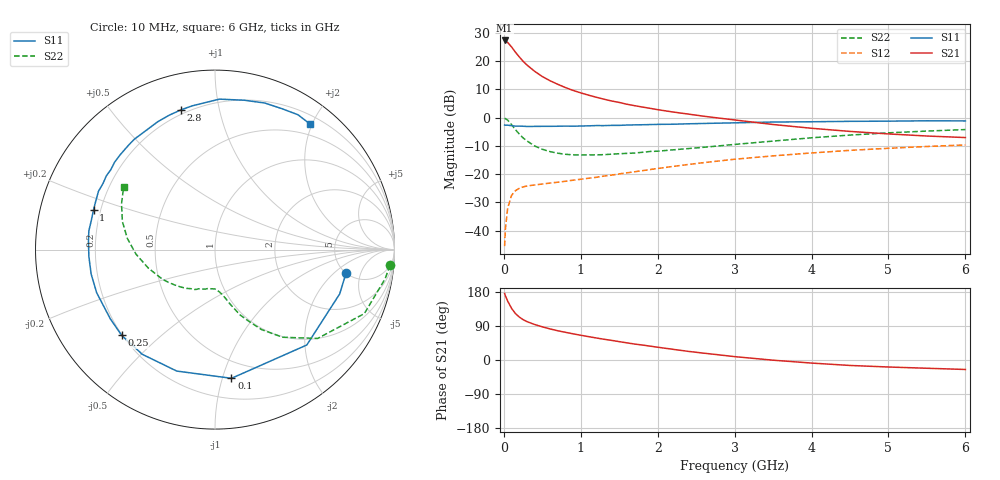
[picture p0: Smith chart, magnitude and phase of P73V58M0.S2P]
! SIEMENS Small Signal Semiconductors
! BFP196
! Si NPN RF Bipolar Junction Transistor in SOT143
! VCE = 3.5 V  IC = 8 mA
! Common Emitter S-Parameters:  May  1996
# GHz  S  MA  R  50
!  f  S11  S21  S12  S22
! GHz  MAG  ANG  MAG  ANG  MAG  ANG  MAG  ANG
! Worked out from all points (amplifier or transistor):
!   36 points, 10 MHz to 6 GHz, reference 50 ohm
!   highest |S21| = 27.4 dB at 10 MHz (marker M1)
!   |S21| within 3 dB of that: start of sweep to 119.2 MHz
!   unconditionally stable (mu >= 1): 947.1 MHz to 3.184 GHz
!   at 250 MHz: K = 0.34, MSG = 22.3 dB, |S12| = -24.5 dB
!   at 1.4 GHz: K = 1.15, MAG = 10.8 dB, |S12| = -20.3 dB
!   at 6 GHz: K = 0.97, MSG = 1.3 dB, |S12| = -9.6 dB
!   S11 on the Smith chart (normalised r, x): 10 MHz: 5.04, -2.89; 100 MHz: 0.36, -1.07; 250 MHz: 0.20, -0.38; 1 GHz: 0.17, +0.16; 2.8 GHz: 0.18, +0.77; 6 GHz: 0.33, +1.98
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0.01  0.7421 -10.0  23.38 175.7  0.0053 86.7  0.9788 -5.1
0.02  0.7372 -19.6  22.89 169.5  0.0106 82.5  0.962 -9.7
0.05  0.7376 -46.1  21.51 155.5  0.0251 68.4  0.9052 -23.2
0.1  0.723 -82.7  17.96 136.4  0.042 52.9  0.7562 -40.9
0.15  0.7095 -107.5  14.52 122.7  0.0509 43.2  0.6163 -52.4
0.2  0.7103 -124.8  11.99 113.5  0.056 37.3  0.5154 -59.8
0.25  0.7061 -137.5  9.997 106.5  0.0595 33.2  0.4398 -64.9
0.3  0.6993 -146.5  8.591 101.4  0.0617 31.9  0.3885 -69.1
0.4  0.7018 -160.0  6.651 93.7  0.0644 29.7  0.3163 -74.4
0.5  0.7034 -168.9  5.366 87.5  0.0669 29.7  0.2759 -78.0
0.6  0.7037 -176.9  4.522 82.1  0.0695 30.3  0.2511 -81.3
0.7  0.7063 176.6  3.913 77.2  0.072 31.4  0.2353 -84.5
0.8  0.7106 171.6  3.429 73.1  0.0748 32.6  0.2251 -87.5
1  0.7124 161.8  2.755 65.3  0.0812 35.3  0.2188 -92.3
1.1  0.7179 157.4  2.513 61.7  0.0846 36.6  0.2194 -95.2
1.6  0.7417 138.9  1.733 45.2  0.1056 40.9  0.2334 -110.0
2.2  0.7667 120.1  1.261 28.2  0.1371 41.6  0.2696 -126.8
2.8  0.8016 103.6  0.984 13.5  0.1716 38.2  0.3173 -144.9
3.5  0.8387 88.3  0.758 -0.5  0.211 31.6  0.3856 -164.5
4.5  0.8625 71.2  0.572 -14.4  0.2642 20.7  0.4925 172.7
5.5  0.8822 58.4  0.474 -21.8  0.3093 9.1  0.5799 153.9
6  0.8773 52.7  0.445 -25.0  0.3294 2.7  0.6169 145.6
